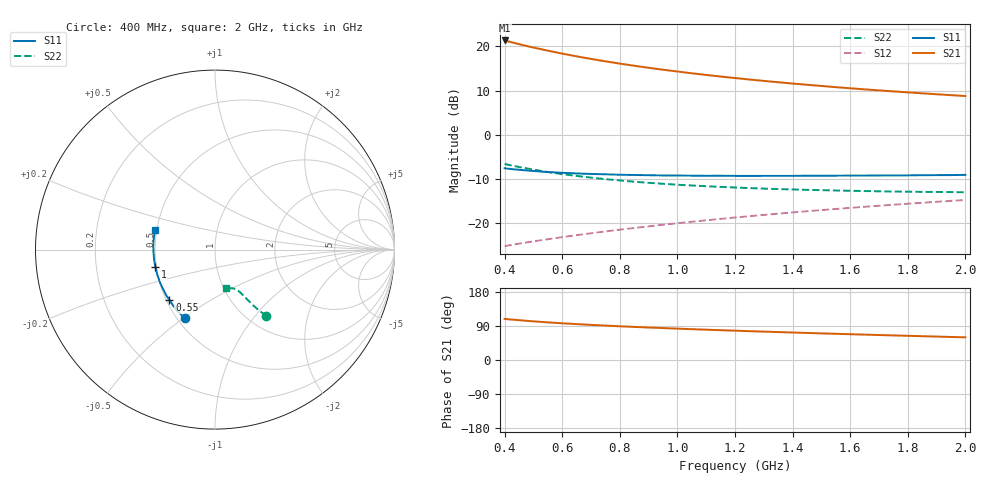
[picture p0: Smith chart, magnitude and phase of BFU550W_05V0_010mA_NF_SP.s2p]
! Filename:  P:\Prog\Test\Noise\ATS_data\Testdata_Net\06 Compressed Noise after Statistics\BFU550W_APM2013_11_D05_05p0V_010mA_NF_CM01_D.sf
! Date/Time: Tue 26/Mar/2013 16:25:22
! BFU550W_APM2013_11_D05_05p0V_1to35mA_NF_CM01_Bias6_R.sf
! Noise Parameter Data File
! BFU550W_APM2013_11_D05_05p0V_1to35mA_NF_CM01
! Date/time: Mon Mar 25 13:26:50 2013
! VAR V_out= 5.000000
! VAR I_out= 10.000000
! VAR V_in= 0.821900
! VAR I_in= 0.103805
! Device data file deembeded for feedlines and parallel
! Original file: \06 Compressed Noise after Statistics\BFU550W_APM2013_11_D05_05p0V_010mA_NF_CM01_R.sf
! Feed-files: PR019V01_070313_Feed1.s2p, PR019V01_070313_Feed2.s2p
! Parallel-file: PR019V01_070313_Par.s2p
# MHz S MA R 50
!  Freq-MHz  S11-mag  S11-arg  S21-mag  S21-arg  S12-mag  S12-arg  S22-mag  S22-arg
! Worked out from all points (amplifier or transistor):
!   37 points, 400 MHz to 2 GHz, reference 50 ohm
!   highest |S21| = 21.3 dB at 400 MHz (marker M1)
!   |S21| within 3 dB of that: start of sweep to 602.5 MHz
!   unconditionally stable (mu >= 1): 1.387 GHz to end of sweep
!   at 500 MHz: K = 0.74, MSG = 21.9 dB, |S12| = -24.1 dB
!   at 1.1 GHz: K = 0.97, MSG = 16.4 dB, |S12| = -19.3 dB
!   at 2 GHz: K = 1.01, MAG = 11.0 dB, |S12| = -14.7 dB
!   lowest NFmin = 0.70 dB at 400 MHz
!   S11 on the Smith chart (normalised r, x): 400 MHz: 0.55, -0.51; 550 MHz: 0.52, -0.34; 1 GHz: 0.49, -0.11; 2 GHz: 0.49, +0.12
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400  0.4173 -113.8  11.64 108.5  0.05504 58.1  0.4669 -52.1
420  0.4108 -116.7  11.19 107.0  0.05657 58.1  0.4527 -52.7
440  0.405 -119.4  10.77 105.7  0.05804 58.2  0.4391 -53.3
460  0.3994 -121.9  10.38 104.4  0.05948 58.4  0.4265 -53.8
500  0.3896 -126.9  9.673 102.0  0.06232 58.6  0.4039 -54.6
550  0.3785 -132.1  8.928 99.3  0.06595 59.1  0.3794 -55.5
600  0.3719 -137.1  8.27 96.9  0.0696 59.6  0.3587 -56.1
650  0.3653 -141.3  7.697 94.7  0.07329 60.0  0.3424 -56.7
700  0.3607 -145.4  7.199 92.7  0.077 60.5  0.3276 -57.3
750  0.3572 -149.0  6.761 90.8  0.08073 61.0  0.315 -57.7
800  0.3533 -152.5  6.372 89.0  0.08454 61.4  0.3046 -58.3
850  0.351 -155.8  6.027 87.3  0.08832 61.7  0.2945 -58.6
950  0.3466 -161.2  5.437 84.2  0.09609 62.4  0.2791 -59.5
1000  0.3461 -163.9  5.185 82.8  0.1 62.6  0.2724 -59.8
1100  0.3438 -168.6  4.744 80.0  0.108 63.1  0.2621 -60.9
1200  0.343 -172.9  4.377 77.4  0.1161 63.3  0.2535 -62.1
1250  0.3427 -175.1  4.212 76.1  0.1201 63.4  0.2495 -62.5
1350  0.343 -178.6  3.923 73.7  0.1284 63.5  0.2432 -63.7
1500  0.3439 176.1  3.559 70.2  0.1408 63.4  0.2366 -65.9
1650  0.3456 171.3  3.261 67.0  0.1534 63.2  0.2312 -68.0
1750  0.3472 168.6  3.092 64.9  0.1619 63.0  0.228 -69.7
2000  0.3519 161.7  2.741 59.8  0.1832 62.0  0.2239 -74.3
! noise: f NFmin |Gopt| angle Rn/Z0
400  0.6977  0.09954  160.2  0.0777
460  0.7209  0.1292  173.4  0.0687
600  0.7542  0.1246  163  0.0743
800  0.7775  0.1583  166.6  0.0692
1000  0.8137  0.1666  169.2  0.069
1200  0.8541  0.1989  172.2  0.0666
1400  0.8838  0.241  177.6  0.0588
1600  0.891  0.2757  -177.1  0.0569
1800  0.9341  0.2916  -174.1  0.0598
2000  0.9642  0.3204  -169  0.0588
